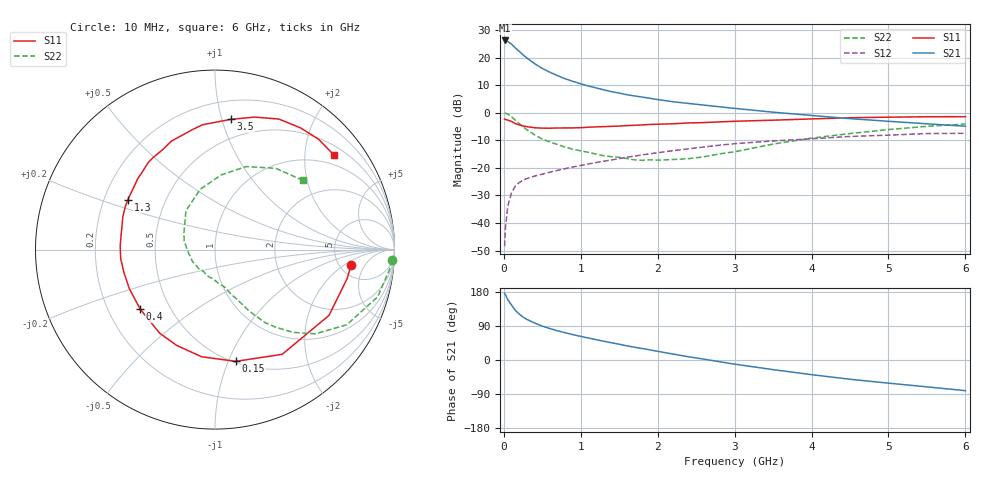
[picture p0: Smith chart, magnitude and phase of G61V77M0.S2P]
! SIEMENS Small Signal Semiconductors
! BFG193
! Si NPN RF Bipolar Junction Transistor in SOT223
! VCE = 1.75 V  IC = 7 mA
! Common Emitter S-Parameters:  August  1996
# GHz  S  MA  R  50
!  f  S11  S21  S12  S22
! GHz  MAG  ANG  MAG  ANG  MAG  ANG  MAG  ANG
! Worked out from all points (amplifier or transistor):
!   36 points, 10 MHz to 6 GHz, reference 50 ohm
!   highest |S21| = 26.2 dB at 10 MHz (marker M1)
!   |S21| within 3 dB of that: start of sweep to 161.7 MHz
!   unconditionally stable (mu >= 1): 971.9 MHz to 2.742 GHz
!   at 250 MHz: K = 0.43, MSG = 22.7 dB, |S12| = -24.5 dB
!   at 1.4 GHz: K = 1.09, MAG = 10.6 dB, |S12| = -17.2 dB
!   at 6 GHz: K = 0.92, MSG = 1.3 dB, |S12| = -7.5 dB
!   S11 on the Smith chart (normalised r, x): 10 MHz: 6.41, -2.58; 150 MHz: 0.51, -1.07; 400 MHz: 0.34, -0.31; 1.3 GHz: 0.30, +0.24; 3.5 GHz: 0.34, +1.07; 6 GHz: 0.72, +2.68
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0.01  0.7639 -6.3  20.39 175.7  0.0038 86.3  0.9862 -3.4
0.02  0.7536 -12.4  20.23 172.6  0.0079 84.3  0.9779 -6.7
0.05  0.7334 -30.0  19.55 160.0  0.0198 74.6  0.9436 -16.2
0.1  0.6932 -57.3  17.47 144.9  0.0357 64.7  0.8453 -29.7
0.15  0.6334 -79.4  14.92 130.9  0.0466 55.2  0.7298 -40.0
0.2  0.6018 -97.1  12.95 121.4  0.0542 50.2  0.6348 -46.6
0.25  0.5747 -111.9  11.19 113.2  0.0596 46.3  0.5489 -52.0
0.3  0.5584 -123.6  9.769 107.0  0.064 44.5  0.4903 -55.7
0.4  0.5326 -141.5  7.754 97.6  0.0709 42.4  0.3955 -60.7
0.5  0.5247 -155.6  6.348 89.3  0.0768 41.4  0.3333 -64.0
0.6  0.5232 -165.8  5.393 82.9  0.0834 41.4  0.2941 -66.9
0.7  0.5278 -174.4  4.684 76.9  0.09 41.7  0.2641 -70.2
0.9  0.5294 171.1  3.684 66.8  0.1038 41.6  0.2174 -75.2
1.1  0.5451 160.4  3.042 58.0  0.1174 41.4  0.191 -83.7
1.3  0.5596 150.2  2.595 49.5  0.1321 40.3  0.1655 -92.1
1.6  0.5839 137.6  2.116 37.3  0.1559 37.2  0.1477 -109.6
2.2  0.6292 117.4  1.58 15.7  0.2049 28.6  0.1416 -152.4
2.8  0.6805 100.6  1.281 -4.4  0.2573 17.5  0.1786 164.1
3.5  0.731 83.1  1.021 -25.4  0.3075 1.7  0.2698 126.9
4.5  0.8098 63.9  0.78 -50.8  0.3707 -18.0  0.4185 85.1
5.5  0.8434 46.8  0.629 -70.9  0.4185 -41.9  0.5655 53.2
6  0.8465 38.6  0.568 -80.9  0.4229 -55.6  0.6226 38.4
